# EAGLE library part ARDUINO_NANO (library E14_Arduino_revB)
Device for representing an Arduino Nano board with a footprint in an EAGLE design. Created by Dave Young for Element14. More EAGLE documentation at: http://www.element14.com/community/community/knode/cadsoft_eagle
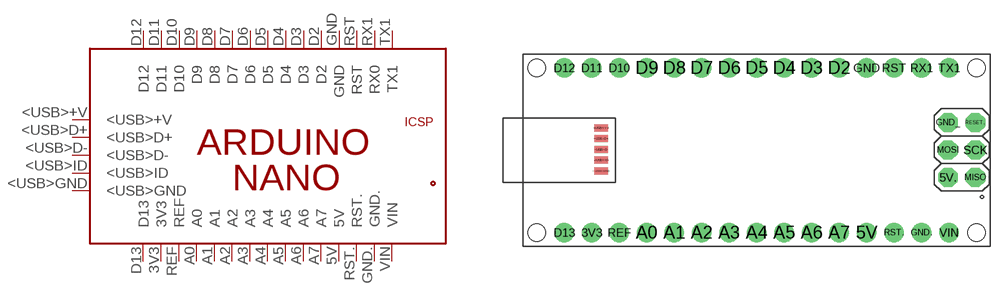
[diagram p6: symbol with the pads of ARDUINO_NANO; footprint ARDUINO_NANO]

Designator prefix PCB

## ARDUINO_NANO  [ARDUINO_NANO]
3V3  3V3
5V  5V
5V.  5V.
<USB>+V  <USB>+V
<USB>D+  <USB>D+
<USB>D-  <USB>D-
<USB>GND  <USB>GND
<USB>ID  <USB>ID
A0  A0
A1  A1
A2  A2
A3  A3
A4  A4
A5  A5
A6  A6
A7  A7
D2  D2
D3  D3
D4  D4
D5  D5
D6  D6
D7  D7
D8  D8
D9  D9
D10  D10
D11  D11
D12  D12
D13  D13
GND  GND
GND.  GND.
GND_  GND_
MISO  MISO
MOSI  MOSI
REF  REF
RESET..  RESET..
RST  RST
RST.  RST.
RX1  RX0
SCK  SCK
TX1  TX1
VIN  VIN

## Footprint ARDUINO_NANO (pad centres in mm)
Footprint for representing an Arduino Nano board in an EAGLE schematic. Created by Dave Young for Element14. More EAGLE documentation at: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
drill 1.016 pad 1.778: 3V3 6.35,1.27; 5V 31.75,1.27; A0 11.43,1.27; A1 13.97,1.27; A2 16.51,1.27; A3 19.05,1.27; A4 21.59,1.27; A5 24.13,1.27; A6 26.67,1.27; A7 29.21,1.27; D2 29.21,16.51; D3 26.67,16.51; D4 24.13,16.51; D5 21.59,16.51; D6 19.05,16.51; D7 16.51,16.51; D8 13.97,16.51; D9 11.43,16.51; D10 8.89,16.51; D11 6.35,16.51; D12 3.81,16.51; D13 3.81,1.27; GND 31.75,16.51; GND. 36.83,1.27; REF 8.89,1.27; RST 34.29,16.51; RST. 34.29,1.27; RX1 36.83,16.51; TX1 39.37,16.51; VIN 39.37,1.27
drill 1.016 pad 1.778 octagon: 5V. 39.268,6.375; GND_ 39.268,11.455; MISO 41.808,6.375; MOSI 39.268,8.915; RESET.. 41.808,11.455; SCK 41.808,8.915
smd 1.27 x 0.635: <USB>+V 7.214,10.947; <USB>D+ 7.214,9.957; <USB>D- 7.214,8.941; <USB>GND 7.214,6.96; <USB>ID 7.214,7.976
hole 1.651 at 1.27,1.27
hole 1.651 at 1.27,16.51
hole 1.651 at 41.91,16.51
hole 1.651 at 41.91,1.27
